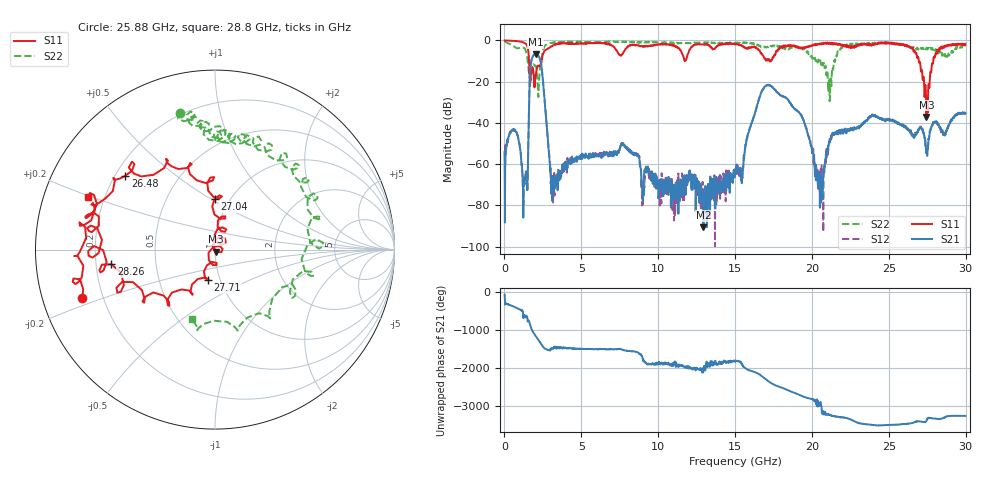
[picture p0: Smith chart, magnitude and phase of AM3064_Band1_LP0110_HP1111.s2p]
# Hz S DB R 50.0
!freq dBS11 angS11 dBS21 angS21 dBS12 angS12 dBS22 angS22
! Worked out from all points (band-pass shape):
!   1600 points, 10 MHz to 29.98 GHz, reference 50 ohm
!   highest |S21| = -6.69 dB at 2.034 GHz (marker M1); lowest = -90.6 dB at 12.94 GHz (marker M2)
!   |S21| within 3 dB of the highest: 1.754 GHz to 2.335 GHz (580.6 MHz wide, 28.4 % of centre)
!   lowest |S11| = -37.1 dB at 27.45 GHz (marker M3), VSWR 1.03, Z = 50.7 - j1.24 ohm
!   |S11| at or under -10 dB: 1.6 GHz to 2.421 GHz (821.5 MHz wide, 40.9 % of centre); 17.24545 GHz to 17.29239 GHz (46.94 MHz wide, 0.272 % of centre); 26.95 GHz to 27.89 GHz (940.3 MHz wide, 3.43 % of centre)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
!   |S22| runs from -29.5 to -0.4 dB; largest |S21 - S12| = 0.0076
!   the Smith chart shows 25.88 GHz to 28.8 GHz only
!   S11 on the Smith chart (normalised r, x): 25.88 GHz: 0.12, -0.18; 26.48 GHz: 0.24, +0.34; 27.04 GHz: 0.85, +0.52; 27.71 GHz: 0.87, -0.31; 28.26 GHz: 0.26, -0.07; 28.8 GHz: 0.14, +0.20
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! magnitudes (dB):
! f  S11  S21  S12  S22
! 10 MHz  0.0  -54.0  -54.0  -0.4
! 1.36 GHz  -1.5  -66.6  -64.0  -4.6
! 1.753 GHz  -14.6  -9.7  -9.7  -17.0
! 2.034 GHz  -16.7  -6.7  -6.6  -12.4
! 3.14 GHz  -2.6  -67.4  -69.3  -1.1
! 5.015 GHz  -1.4  -55.2  -56.4  -0.6
! 10 GHz  -2.1  -68.2  -67.5  -1.0
! 12.94 GHz  -2.0  -90.6  -79.2  -1.1
! 15 GHz  -1.8  -63.5  -62.1  -1.3
! 17.09 GHz  -9.1  -21.7  -21.8  -3.1
! 19.99 GHz  -2.8  -52.4  -52.2  -8.2
! 20.53 GHz  -1.6  -69.3  -66.0  -9.6
! 21.45 GHz  -2.0  -45.8  -45.5  -9.7
! 25 GHz  -1.0  -38.4  -38.5  -1.3
! 25.88 GHz  -2.1  -40.8  -41.1  -2.1
! 26.48 GHz  -3.8  -44.9  -44.6  -3.4
! 27.04 GHz  -11.0  -42.0  -42.5  -4.5
! 27.45 GHz  -37.1  -54.6  -54.8  -3.6
! 27.71 GHz  -15.2  -43.1  -43.0  -3.6
! 28.26 GHz  -4.7  -41.3  -41.4  -5.7
! 28.8 GHz  -2.3  -42.9  -42.4  -7.8
! 29.98 GHz  -1.7  -35.4  -35.5  -3.0
